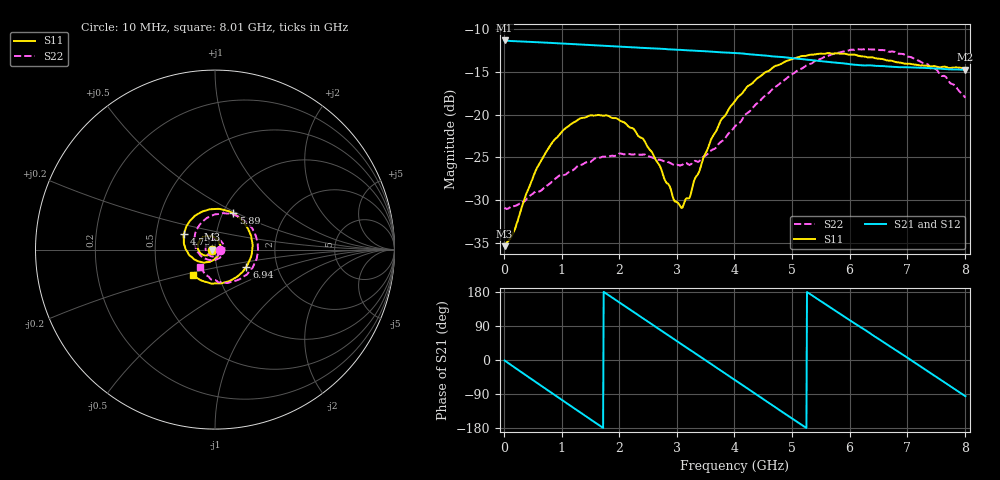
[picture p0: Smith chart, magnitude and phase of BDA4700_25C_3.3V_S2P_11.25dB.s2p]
!Agilent Technologies,E5071B,MY42404982,A.09.10
!Date: Mon Oct 20 18:07:44 2025
!Data & Calibration Information:
!Freq	S11:SOLT2(ON)	S21:SOLT2(ON)	S12:SOLT2(ON)	S22:SOLT2(ON)
# Hz S RI R 50
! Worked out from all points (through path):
!   801 points, 10 MHz to 8.01 GHz, reference 50 ohm
!   highest |S21| = -11.36 dB at 10 MHz (marker M1); lowest = -14.8 dB at 8.01 GHz (marker M2)
!   group delay of S21, straight-line fit = 282 ps
!   lowest |S11| = -35.4 dB at 10 MHz (marker M3), VSWR 1.03, Z = 48.3 - j0.106 ohm
!   |S11| at or under -10 dB: start of sweep to end of sweep
!   |S22| runs from -31.0 to -12.4 dB; largest |S21 - S12| = 0.003
!   S11 on the Smith chart (normalised r, x): 10 MHz: 0.97, -0.00; 4.75 GHz: 0.70, +0.13; 5.89 GHz: 1.12, +0.48; 6.94 GHz: 1.39, -0.27; 8.01 GHz: 0.75, -0.22
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1e7  -0.017 -0.00109  0.2703 -0.00601  0.2703 -0.00609  0.0286 -0.00146
1.6e8  -0.0179 -0.0097  0.256 -0.0792  0.256 -0.0792  0.0276 -0.0094
5.3e8  -0.0348 -0.0292  0.1481 -0.2191  0.1479 -0.2192  0.0136 -0.0325
7.2e8  -0.0496 -0.0329  0.0644 -0.2544  0.0647 -0.2545  -0.00173 -0.0379
1.02e9  -0.077 -0.0236  -0.0753 -0.2483  -0.0754 -0.2484  -0.0286 -0.0339
1.35e9  -0.0953 0.00588  -0.1992 -0.161  -0.1992 -0.1612  -0.0506 -0.00644
1.93e9  -0.0676 0.0673  -0.2336 0.0889  -0.2335 0.0889  -0.0267 0.0508
2.26e9  -0.0282 0.0767  -0.1424 0.2009  -0.1426 0.2009  0.0113 0.0574
2.68e9  0.019 0.0481  0.0316 0.2401  0.0312 0.2399  0.0485 0.0249
2.96e9  0.0294 0.0103  0.1404 0.1935  0.1402 0.1932  0.0502 -0.00896
3.1e9  0.0269 -0.01  0.1834 0.1513  0.1822 0.1525  0.0437 -0.0267
3.54e9  -0.0164 -0.0614  0.2325 -0.0204  0.2325 -0.0207  -0.00574 -0.0588
4.01e9  -0.1034 -0.0608  0.1373 -0.1825  0.1376 -0.182  -0.0763 -0.0378
4.38e9  -0.161 -0.00249  -0.00307 -0.2231  -0.00316 -0.2233  -0.113 0.0226
4.75e9  -0.1724 0.0879  -0.136 -0.1694  -0.1352 -0.1703  -0.1045 0.1045
5.35e9  -0.0641 0.2142  -0.2044 0.0348  -0.2046 0.0336  0.0193 0.1983
5.89e9  0.1013 0.2024  -0.0875 0.1785  -0.0878 0.1779  0.1742 0.1542
6.29e9  0.1868 0.1094  0.043 0.1884  0.0453 0.1872  0.2367 0.0424
6.68e9  0.2055 -0.0169  0.1499 0.1171  0.1504 0.1169  0.2195 -0.0774
6.94e9  0.1749 -0.0943  0.1842 0.0404  0.1844 0.0393  0.1742 -0.1414
7.47e9  0.0353 -0.1882  0.1404 -0.1217  0.1403 -0.122  0.0244 -0.1829
8.01e9  -0.1221 -0.1421  -0.0178 -0.1815  -0.0174 -0.1816  -0.0826 -0.0943
